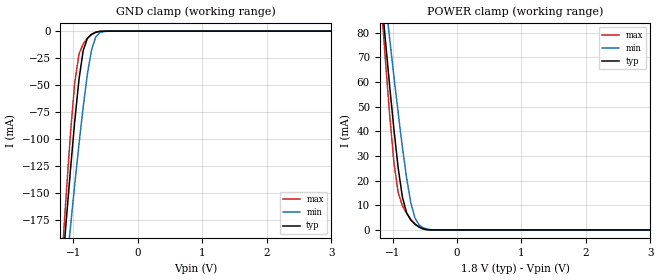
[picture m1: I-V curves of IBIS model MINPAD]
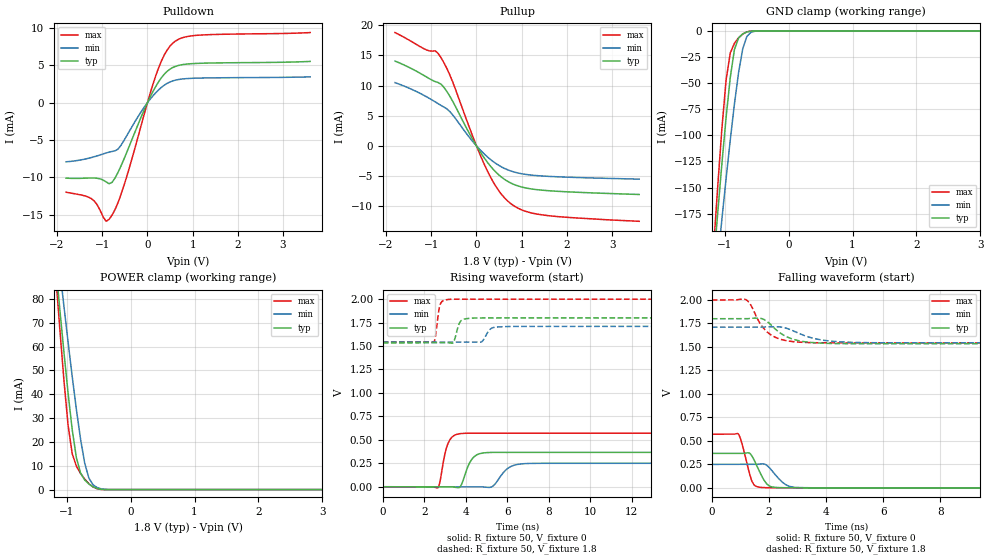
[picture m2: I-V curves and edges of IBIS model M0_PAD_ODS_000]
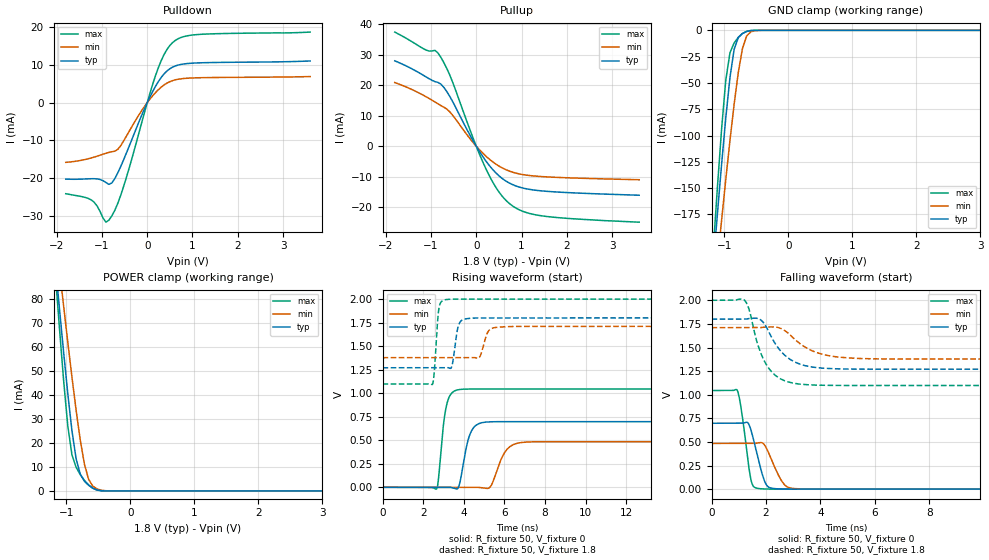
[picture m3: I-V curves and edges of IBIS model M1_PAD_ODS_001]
|   Microsemi Corporation
|   SmartFusion2 Automotive IBIS Model
[IBIS ver]   5.0
[File name]   as30208cc_18v_rev2p12.ibs
[File Rev]   2.12
[Date]   Wed Apr 02 2025
[Source] Simulated Models ONLY.
   All data is based on Spice simulation. All performed at Microsemi Corporation.
   Please refer to the Microsemi website for future updates at www.microsemi.com
[Notes]  Microsemi SmartFusion2 IBIS models for automotive operating conditions
   for DDRIO IO Banks IO Configurations ONLY. Models uses a software default
   fixed codes except for DDR3/SSTL15 which will always require calibrated
   codes.
   Automotive Temperature Grade 2 (t2) models cover a temperature range from
   -40C to 125C.
   Please refer to msio_auto_t2.ibs for MSIO IO Banks IO Configurations.
   Please refer to msiod_auto_t2.ibs for MSIOD IO Banks IO Configurations.
   The package parasitics of various package types are given.
   Uncomment the appropriate package or refer to the .pkg for specific
   per pin parasitic data.
   There are warnings related to non-monotonic and Increasing/Decreasing Current.
   They are expected on 20 Ohms and 30 Ohms I/O ODT models in DDR3/SSTL15.
[Disclaimer] This information is for board design considerations.
   Simulation based V/I curves contained in this model file are
   considered preliminary until verified against bench
   measurements. Maximum currents may vary from part to part but
   should not exceed maximum I/V curves provided in this model file.
[Copyright]  (c) 2015, Microsemi Corporation, All Rights Reserved.
| IBIS MODEL CHECKLIST
| Microsemi is dedicated to releasing quality IBIS models to customers.
| The following items have been
| verified for this IBIS model before release:
| 1)  Checked IBIS model by the golden parser ibischk5 [Complete]
| 2)  Ensured no errors reported by golden parser
|   for the IBIS model [Complete]
| 3)  Defined Vinl and Vinh for recievers [Complete]
| 4)  Defined Standard Load and Vmeas values for drivers [Complete]
| 5)  Defined overshoots for drivers and recievers [NA]
| 6)  Validated Ramp Values[Complete]
| 7)  Defined V-T Tables for all output drivers [Complete]
| 8)  Validated [Diff Pins] []
| 9)  Verified Package Parasitics [Complete]
| 10) Defined Standard Load Parameters and Specifications
|   for waveforms [Complete]
| 11) Defined and Validate Pin mappings [Complete]
| 12) Verified Ccomp Value []
| 13) Visually Inspected I-V Curves and V-T Tables  [Complete]
| 14) Presented Typ/Min/Max Values in the correct order for
|   all tables and parameters [Complete]
| 15) Simulated all output models with standard load and
|   switching through Vmeas [Complete]
| 16) Simulated all reciever models  [Complete]
| 17) Validated Models selectors. []
| 18) Visually inspected Spice and IBIS correlation for
|   a) Typical VT Curves [Complete]
|   b) Minimum VT Curves [Complete]
|   c) Maximum VT Curves [Complete]
| 19) Visually inspected Silicon and IBIS correlation
|   a) Typical IV Pull UP/ Pull Down Curves []
|   b) Minimum IV Pull UP/ Pull Down Curves []
|   c) Maximum IV Pull UP/ Pull Down Curves []
|   Component SmartFusion2
[Component]   SmartFusion2 W MRAM
[Manufacturer]   Avalanche Technology
[Package]
|  Design die-package: BGA
| variable   typ   min   max
R_pkg   0.72029   0.51528   1.0002
L_pkg   5.797e-9   4.155e-9   8.073e-9
C_pkg   1.116e-12   7.907e-13   1.753e-12
|Pin and Model info
[Pin]  signal_name  model_name   R_pin   L_pin   C_pin
L7   CS1#   MINPAD   0.4340		15.2000E-9		1.2600E-12
J8   CS2#   MINPAD   0.3800		13.5000E-9		1.0400E-12
K7   CLK1   MINPAD   0.4300		12.7000E-9		0.9790E-12
K6   CLK2   MINPAD   0.4480		14.6000E-9		1.1600E-12
M8   IO_0   MIOPAD   0.4010		12.4000E-9		1.2500E-12
M7   IO_1   MIOPAD   0.4050		14.2000E-9		1.1100E-12
L9   IO_2   MIOPAD   0.3780		11.8000E-9		1.2000E-12
M9   IO_3   MIOPAD   0.3700		11.8000E-9		1.2600E-12
M10   IO_4   MIOPAD   0.3710		11.1000E-9		1.1000E-12
N8   IO_5   MIOPAD   0.4050		13.8000E-9		1.1600E-12
N7   IO_6   MIOPAD   0.3830		15.2000E-9		1.0900E-12
N6   IO_7   MIOPAD   0.4480		16.4000E-9		1.0800E-12
J12   HTBSEL   MINPAD   0.1380		6.1700E-9		0.6060E-12
H12   HBP_2   MINPAD   0.1470		6.3900E-9		1.0000E-12
G11   HBP_1   MINPAD   0.1910		8.5000E-9		1.1500E-12
G10   HBP_0   MINPAD   0.2050		8.6800E-9		1.4200E-12
J9   RESET#   MINPAD   0.3410		14.1000E-9		1.6300E-12
J10   INT1#   MIOPAD   0.3080		12.5000E-9		1.2100E-12
K8   INT2#   MIOPAD   0.2120		10.3000E-9		0.8230E-12
M5   VSSIO   GND   NA   NA   NA
H6   VSSIO   GND   NA   NA   NA
L6   VSSIO   GND   NA   NA   NA
P8   VSSIO   GND   NA   NA   NA
H10   VSSIO   GND   NA   NA   NA
N10   VSSIO   GND   NA   NA   NA
P10   VSSIO   GND   NA   NA   NA
H11   VSSIO   GND   NA   NA   NA
N11   VSSIO   GND   NA   NA   NA
A1   VSS   GND   NA   NA   NA
B1   VSS   GND   NA   NA   NA
W1   VSS   GND   NA   NA   NA
Y1   VSS   GND   NA   NA   NA
A2   VSS   GND   NA   NA   NA
Y2   VSS   GND   NA   NA   NA
F3   VSS   GND   NA   NA   NA
G3   VSS   GND   NA   NA   NA
P3   VSS   GND   NA   NA   NA
R3   VSS   GND   NA   NA   NA
F4   VSS   GND   NA   NA   NA
H4   VSS   GND   NA   NA   NA
J4   VSS   GND   NA   NA   NA
L4   VSS   GND   NA   NA   NA
N4   VSS   GND   NA   NA   NA
R4   VSS   GND   NA   NA   NA
L5   VSS   GND   NA   NA   NA
N5   VSS   GND   NA   NA   NA
G6   VSS   GND   NA   NA   NA
P6   VSS   GND   NA   NA   NA
G8   VSS   GND   NA   NA   NA
H8   VSS   GND   NA   NA   NA
L10   VSS   GND   NA   NA   NA
L11   VSS   GND   NA   NA   NA
P11   VSS   GND   NA   NA   NA
F12   VSS   GND   NA   NA   NA
L12   VSS   GND   NA   NA   NA
N12   VSS   GND   NA   NA   NA
R12   VSS   GND   NA   NA   NA
F13   VSS   GND   NA   NA   NA
G13   VSS   GND   NA   NA   NA
P13   VSS   GND   NA   NA   NA
R13   VSS   GND   NA   NA   NA
A14   VSS   GND   NA   NA   NA
Y14   VSS   GND   NA   NA   NA
A15   VSS   GND   NA   NA   NA
B15   VSS   GND   NA   NA   NA
W15   VSS   GND   NA   NA   NA
Y15   VSS   GND   NA   NA   NA
G4   VCCIO   POWER   NA   NA   NA
P4   VCCIO   POWER   NA   NA   NA
G5   VCCIO   POWER   NA   NA   NA
J5   VCCIO   POWER   NA   NA   NA
P5   VCCIO   POWER   NA   NA   NA
M6   VCCIO   POWER   NA   NA   NA
H7   VCCIO   POWER   NA   NA   NA
H9   VCCIO   POWER   NA   NA   NA
N9   VCCIO   POWER   NA   NA   NA
J11   VCCIO   POWER   NA   NA   NA
M11   VCCIO   POWER   NA   NA   NA
G12   VCCIO   POWER   NA   NA   NA
P12   VCCIO   POWER   NA   NA   NA
K4   VCC   POWER   NA   NA   NA
M4   VCC   POWER   NA   NA   NA
K5   VCC   POWER   NA   NA   NA
G7   VCC   POWER   NA   NA   NA
P7   VCC   POWER   NA   NA   NA
G9   VCC   POWER   NA   NA   NA
K9   VCC   POWER   NA   NA   NA
P9   VCC   POWER   NA   NA   NA
K11   VCC   POWER   NA   NA   NA
K12   VCC   POWER   NA   NA   NA
M12   VCC   POWER   NA   NA   NA
| END PIN INFO
| IOPAD
[Model Selector] MIOPAD
| Model Description
M0_PAD_ODS_000   ODS_000
M1_PAD_ODS_001   ODS_001
M2_PAD_ODS_010   ODS_010
M3_PAD_ODS_011   ODS_011
M4_PAD_ODS_100   ODS_100
M5_PAD_ODS_101   ODS_101
M6_PAD_ODS_110   ODS_110
M7_PAD_ODS_111   ODS_111
| Models and submodels in the file (9): MINPAD (Input), M0_PAD_ODS_000 (I/O), M1_PAD_ODS_001 (I/O), M2_PAD_ODS_010 (I/O), M3_PAD_ODS_011 (I/O), M4_PAD_ODS_100 (I/O), M5_PAD_ODS_101 (I/O), M6_PAD_ODS_110 (I/O), M7_PAD_ODS_111 (I/O)
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[Model] MINPAD
Model_type Input
Enable   Active-High
Vinl  =  0.63
Vinh  =  1.17
| Capacitance  typ   min   max
C_comp   1.624351e-12   1.517192e-12   1.739751e-12
| Variables   typ   min   max
[GND Clamp Reference]   0   0   0
[POWER Clamp Reference]   1.8   1.71   2
[Pulldown Reference]   0   0   0
[Pullup Reference]   1.8   1.71   2
[Temperature Range]   25   125   -40
[Voltage Range]   1.8   1.71   2
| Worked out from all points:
|   GND clamp passes 1 mA (typ) near -0.64 V on its own axis
|   POWER clamp passes 1 mA (typ) near -0.57 V on its own axis
[GND Clamp]
| Voltage   I(typ)   I(min)   I(max)
-1.8V     -720.5mA   -670.5mA   -825.4mA
-1.173V   -222.3mA   -260.3mA   -207.7mA
-1.108V   -173.8mA   -219.8mA   -148.5mA
-1.043V   -127mA     -180.1mA   -93.29mA
-977.6mV  -83.06mA   -141.5mA   -47.18mA
-912.4mV  -44.72mA   -104.6mA   -21.22mA
-847.2mV  -17.98mA   -70.1mA    -11.91mA
-782.1mV  -6.764mA   -39.85mA   -6.651mA
-716.9mV  -2.937mA   -17.13mA   -3.044mA
-651.7mV  -1.118mA   -5.25mA    -949.8uA
-456.2mV  -3.975uA   -74.4uA    -419.6nA
3.6V      0A         0A         0A
[POWER Clamp]
| Voltage   I(typ)   I(min)   I(max)
-1.8V     287.1mA    268.3mA    329.6mA
-1.173V   94.89mA    108.5mA    91.02mA
-1.108V   76.1mA     92.66mA    67.97mA
-1.043V   57.9mA     77.16mA    46.14mA
-977.6mV  40.62mA    62.05mA    27.14mA
-912.4mV  25.13mA    47.46mA    15.06mA
-847.2mV  13.38mA    33.64mA    9.853mA
-716.9mV  4.014mA    11.09mA    4.394mA
-651.7mV  2.34mA     4.821mA    2.483mA
-586.6mV  1.18mA     2.003mA    1.113mA
-325.9mV  1.153uA    19.85uA    110.1nA
3.6V      0A         0A         0A
[Model] M0_PAD_ODS_000
Model_type I/O
Enable   Active-High
Vinl  =  0.63
Vinh  =  1.17
Vmeas =  0.9
Cref  =  30e-12
| Capacitance  typ   min   max
C_comp   1.627116e-12   1.521588e-12   1.744735e-12
| Variables   typ   min   max
[GND Clamp Reference]   0   0   0
[POWER Clamp Reference]   1.8   1.71   2
[Pulldown Reference]   0   0   0
[Pullup Reference]   1.8   1.71   2
[Temperature Range]   25   125   -40
[Voltage Range]   1.8   1.71   2
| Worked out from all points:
|   slope of the pulldown table from 0 to 0.27 V, typ, clamps not added: 89.8 ohm
|   slope of the pullup table from 0 to 0.27 V, typ, clamps not added: 90.4 ohm
|   GND clamp passes 1 mA (typ) near -0.64 V on its own axis
|   POWER clamp passes 1 mA (typ) near -0.57 V on its own axis
|   falling waveform, R_fixture 50, V_fixture 0: 20-80 % time 364ps typ, 459ps min, 289ps max; typ from 0.367 V to 0 V
|   falling waveform, R_fixture 50, V_fixture 1.8: 20-80 % time 770ps typ, 991ps min, 610ps max; typ from 1.8 V to 1.53 V
|   rising waveform, R_fixture 50, V_fixture 0: 20-80 % time 416ps typ, 570ps min, 332ps max; typ from 0 V to 0.367 V
|   rising waveform, R_fixture 50, V_fixture 1.8: 20-80 % time 213ps typ, 281ps min, 164ps max; typ from 1.53 V to 1.8 V
[GND Clamp]
| Voltage   I(typ)   I(min)   I(max)
-1.8V     -720.5mA   -670.5mA   -825.4mA
-1.173V   -222.3mA   -260.3mA   -207.7mA
-1.108V   -173.8mA   -219.8mA   -148.5mA
-1.043V   -127mA     -180.1mA   -93.3mA
-977.6mV  -83.06mA   -141.5mA   -47.19mA
-912.4mV  -44.72mA   -104.6mA   -21.23mA
-847.2mV  -17.99mA   -70.1mA    -11.92mA
-782.1mV  -6.766mA   -39.85mA   -6.657mA
-716.9mV  -2.938mA   -17.13mA   -3.048mA
-651.7mV  -1.119mA   -5.25mA    -952uA
-456.2mV  -3.98uA    -74.41uA   -422.2nA
3.6V      0A         0A         0A
[POWER Clamp]
| Voltage   I(typ)   I(min)   I(max)
-1.8V     287.1mA    268.3mA    329.6mA
-1.173V   94.89mA    108.5mA    91.02mA
-1.108V   76.1mA     92.66mA    67.97mA
-1.043V   57.9mA     77.16mA    46.14mA
-977.6mV  40.62mA    62.05mA    27.14mA
-912.4mV  25.13mA    47.46mA    15.06mA
-847.2mV  13.38mA    33.64mA    9.853mA
-716.9mV  4.014mA    11.09mA    4.394mA
-651.7mV  2.34mA     4.821mA    2.483mA
-586.6mV  1.18mA     2.003mA    1.113mA
-325.9mV  1.153uA    19.85uA    110.1nA
3.6V      0A         0A         0A
[Pulldown]
| Voltage   I(typ)   I(min)   I(max)
-1.8V     -10.09mA   -7.898mA   -11.97mA
-1.238V   -10.07mA   -7.328mA   -12.83mA
-912.4mV  -10.59mA   -6.717mA   -15.86mA
-847.2mV  -10.83mA   -6.605mA   -15.6mA
-716.9mV  -10.08mA   -6.431mA   -14.3mA
-521.4mV  -7.575mA   -5.077mA   -11.12mA
-65.17mV  -872uA     -545.4uA   -1.404mA
248.3mV   2.817mA    1.73mA     4.683mA
434.5mV   4.193mA    2.586mA    7.041mA
620.7mV   4.869mA    3.026mA    8.258mA
1.179V    5.284mA    3.307mA    9.058mA
3.6V      5.531mA    3.462mA    9.391mA
[Pullup]
| Voltage   I(typ)   I(min)   I(max)
-1.8V     14.07mA    10.49mA    18.8mA
-1.108V   11.45mA    8.161mA    15.93mA
-912.4mV  10.66mA    7.301mA    15.78mA
-782.1mV  10.22mA    6.706mA    14.62mA
-586.6mV  8.214mA    5.673mA    11.74mA
-65.17mV  835.7uA    571.5uA    1.251mA
248.3mV   -2.782mA   -1.866mA   -4.251mA
496.6mV   -4.831mA   -3.242mA   -7.473mA
744.8mV   -6.111mA   -4.126mA   -9.499mA
1.055V    -6.927mA   -4.698mA   -10.78mA
1.428V    -7.337mA   -4.986mA   -11.42mA
3.6V      -8.069mA   -5.52mA    -12.52mA
[Ramp]
dV/dt_r   0.220223/0.415702n  0.150081/0.569672n  0.34276/0.331988n
dV/dt_f   0.159898/0.770039n  0.100158/0.991323n  0.274318/0.609698n
R_load = 50
[Falling Waveform]
R_fixture = 50
V_fixture = 0
V_fixture_min = 0
V_fixture_max = 0
| Time   V(typ)   V(min)   V(max)
0s        367mV      250.1mV    571.3mV
923.8ps   367.3mV    250.7mV    573.7mV
1.037ns   367.3mV    250.7mV    489.3mV
1.291ns   372.9mV    250.9mV    184mV
1.42ns    330.5mV    250.9mV    60.14mV
1.744ns   128.3mV    254.8mV    4.316mV
2.055ns   13.67mV    200.4mV    1.169mV
2.601ns   1.34mV     30.95mV    220.5uV
2.98ns    480.5uV    4.171mV    216.1uV
21.88ns   3.869uV    78.26nV    -3.43uV
[Falling Waveform]
R_fixture = 50
V_fixture = 1.8
V_fixture_min = 1.71
V_fixture_max = 2
| Time   V(typ)   V(min)   V(max)
0s        1.8V       1.71V      2V
1.194ns   1.801V     1.71V      2.003V
1.367ns   1.805V     1.71V      1.943V
1.68ns    1.806V     1.711V     1.755V
1.949ns   1.766V     1.714V     1.656V
2.444ns   1.638V     1.711V     1.578V
2.887ns   1.578V     1.666V     1.554V
3.81ns    1.541V     1.576V     1.544V
5.079ns   1.534V     1.547V     1.543V
21.88ns   1.534V     1.543V     1.543V
[Rising Waveform]
R_fixture = 50
V_fixture = 0
V_fixture_min = 0
V_fixture_max = 0
| Time   V(typ)   V(min)   V(max)
0s        3.036nV    85.33nV    -62.8nV
2.644ns   -691.4uV   -545.1uV   -11.75mV
3.145ns   -822.4uV   -648.4uV   462.5mV
3.72ns    -1.25mV    -766.9uV   565.8mV
4.314ns   300mV      -889.5uV   570.7mV
5.019ns   364.1mV    -5.657mV   570.7mV
5.313ns   366.1mV    6.668mV    570.7mV
6.157ns   366.1mV    214mV      570.8mV
6.888ns   366.1mV    247mV      570.8mV
21.88ns   367mV      250.1mV    571.3mV
[Rising Waveform]
R_fixture = 50
V_fixture = 1.8
V_fixture_min = 1.71
V_fixture_max = 2
| Time   V(typ)   V(min)   V(max)
0s        1.534V     1.543V     1.543V
2.445ns   1.534V     1.543V     1.54V
2.53ns    1.534V     1.543V     1.594V
2.745ns   1.534V     1.543V     1.929V
3.139ns   1.534V     1.543V     1.996V
3.396ns   1.538V     1.543V     1.999V
3.757ns   1.766V     1.543V     1.999V
4.265ns   1.797V     1.543V     1.999V
5.688ns   1.8V       1.705V     1.999V
21.88ns   1.8V       1.71V      2V
[Model] M1_PAD_ODS_001
Model_type I/O
Enable   Active-High
Vinl  =  0.63
Vinh  =  1.17
Vmeas =  0.9
Cref  =  30e-12
| Capacitance  typ   min   max
C_comp   1.627116e-12   1.521588e-12   1.744735e-12
| Variables   typ   min   max
[GND Clamp Reference]   0   0   0
[POWER Clamp Reference]   1.8   1.71   2
[Pulldown Reference]   0   0   0
[Pullup Reference]   1.8   1.71   2
[Temperature Range]   25   125   -40
[Voltage Range]   1.8   1.71   2
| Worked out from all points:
|   slope of the pulldown table from 0 to 0.27 V, typ, clamps not added: 44.9 ohm
|   slope of the pullup table from 0 to 0.27 V, typ, clamps not added: 45.3 ohm
|   GND clamp passes 1 mA (typ) near -0.64 V on its own axis
|   POWER clamp passes 1 mA (typ) near -0.57 V on its own axis
|   falling waveform, R_fixture 50, V_fixture 0: 20-80 % time 370ps typ, 463ps min, 286ps max; typ from 0.698 V to 0 V
|   falling waveform, R_fixture 50, V_fixture 1.8: 20-80 % time 821ps typ, 1.04ns min, 652ps max; typ from 1.8 V to 1.27 V
|   rising waveform, R_fixture 50, V_fixture 0: 20-80 % time 411ps typ, 571ps min, 311ps max; typ from 0 V to 0.698 V
|   rising waveform, R_fixture 50, V_fixture 1.8: 20-80 % time 216ps typ, 282ps min, 166ps max; typ from 1.27 V to 1.8 V
[GND Clamp]
| Voltage   I(typ)   I(min)   I(max)
-1.8V     -720.5mA   -670.5mA   -825.4mA
-1.173V   -222.3mA   -260.3mA   -207.7mA
-1.108V   -173.8mA   -219.8mA   -148.5mA
-1.043V   -127mA     -180.1mA   -93.3mA
-977.6mV  -83.06mA   -141.5mA   -47.19mA
-912.4mV  -44.72mA   -104.6mA   -21.23mA
-847.2mV  -17.99mA   -70.1mA    -11.92mA
-782.1mV  -6.766mA   -39.85mA   -6.657mA
-716.9mV  -2.938mA   -17.13mA   -3.048mA
-651.7mV  -1.119mA   -5.25mA    -952uA
-456.2mV  -3.98uA    -74.41uA   -422.2nA
3.6V      0A         0A         0A
[POWER Clamp]
| Voltage   I(typ)   I(min)   I(max)
-1.8V     287.1mA    268.3mA    329.6mA
-1.173V   94.89mA    108.5mA    91.02mA
-1.108V   76.1mA     92.66mA    67.97mA
-1.043V   57.9mA     77.16mA    46.14mA
-977.6mV  40.62mA    62.05mA    27.14mA
-912.4mV  25.13mA    47.46mA    15.06mA
-847.2mV  13.38mA    33.64mA    9.853mA
-716.9mV  4.014mA    11.09mA    4.394mA
-651.7mV  2.34mA     4.821mA    2.483mA
-586.6mV  1.18mA     2.003mA    1.113mA
-325.9mV  1.153uA    19.85uA    110.1nA
3.6V      0A         0A         0A
[Pulldown]
| Voltage   I(typ)   I(min)   I(max)
-1.8V     -20.26mA   -15.83mA   -24.15mA
-1.238V   -20.17mA   -14.67mA   -25.78mA
-912.4mV  -21.17mA   -13.42mA   -31.69mA
-847.2mV  -21.66mA   -13.2mA    -31.16mA
-716.9mV  -20.14mA   -12.86mA   -28.56mA
-521.4mV  -15.14mA   -10.15mA   -22.2mA
-65.17mV  -1.742mA   -1.091mA   -2.802mA
248.3mV   5.63mA     3.46mA     9.353mA
434.5mV   8.383mA    5.171mA    14.07mA
620.7mV   9.735mA    6.051mA    16.51mA
1.179V    10.57mA    6.614mA    18.12mA
3.6V      11.06mA    6.923mA    18.71mA
[Pullup]
| Voltage   I(typ)   I(min)   I(max)
-1.8V     28.03mA    20.89mA    37.45mA
-1.108V   22.74mA    16.24mA    31.55mA
-912.4mV  21.2mA     14.52mA    31.47mA
-782.1mV  20.39mA    13.35mA    29.17mA
-521.4mV  14.66mA    10.17mA    21.02mA
-130.3mV  3.403mA    2.332mA    5.058mA
186.2mV   -4.285mA   -2.877mA   -6.521mA
496.6mV   -9.629mA   -6.461mA   -14.9mA
744.8mV   -12.18mA   -8.22mA    -18.94mA
1.055V    -13.81mA   -9.36mA    -21.49mA
1.49V     -14.71mA   -9.993mA   -22.92mA
3.6V      -16.07mA   -10.99mA   -24.92mA
[Ramp]
dV/dt_r   0.418626/0.410816n  0.290552/0.571412n  0.626829/0.311374n
dV/dt_f   0.317973/0.820722n  0.199636/1.04338n  0.541445/0.651669n
R_load = 50
[Falling Waveform]
R_fixture = 50
V_fixture = 0
V_fixture_min = 0
V_fixture_max = 0
| Time   V(typ)   V(min)   V(max)
0s        697.7mV    484.3mV    1.045V
951.4ps   698.1mV    484.5mV    1.042V
1.108ns   698.1mV    484.5mV    814.4mV
1.331ns   703.6mV    484.6mV    322mV
1.452ns   622mV      484.6mV    93.29mV
1.73ns    303.2mV    490.6mV    6.618mV
2.068ns   27.7mV     403mV      1.399mV
2.572ns   2.158mV    87.65mV    450.6uV
3.037ns   658.8uV    6.568mV    439.8uV
21.88ns   1.498nV    129.2nV    255.6nV
[Falling Waveform]
R_fixture = 50
V_fixture = 1.8
V_fixture_min = 1.71
V_fixture_max = 2
| Time   V(typ)   V(min)   V(max)
0s        1.8V       1.71V      2V
1.215ns   1.801V     1.71V      2V
1.378ns   1.807V     1.71V      1.904V
1.7ns     1.808V     1.71V      1.529V
1.992ns   1.728V     1.717V     1.329V
2.553ns   1.458V     1.701V     1.165V
3.071ns   1.345V     1.583V     1.119V
4.039ns   1.282V     1.431V     1.1V
5.423ns   1.271V     1.384V     1.098V
21.88ns   1.27V      1.377V     1.098V
[Rising Waveform]
R_fixture = 50
V_fixture = 0
V_fixture_min = 0
V_fixture_max = 0
| Time   V(typ)   V(min)   V(max)
0s        2.474nV    66.45nV    166.5nV
2.668ns   -425.3uV   -220uV     -14.74mV
3.141ns   -500.7uV   -259uV     861mV
3.645ns   -17.16mV   -300.5uV   1.033V
4.267ns   540.5mV    -351.8uV   1.044V
4.874ns   685.9mV    -4.978mV   1.044V
5.31ns    695.8mV    6.141mV    1.044V
6.12ns    697mV      401.5mV    1.044V
6.901ns   697.1mV    477.2mV    1.044V
21.88ns   697.7mV    484.3mV    1.045V
[Rising Waveform]
R_fixture = 50
V_fixture = 1.8
V_fixture_min = 1.71
V_fixture_max = 2
| Time   V(typ)   V(min)   V(max)
0s        1.27V      1.377V     1.098V
2.449ns   1.271V     1.378V     1.092V
2.769ns   1.271V     1.378V     1.892V
3.098ns   1.271V     1.378V     1.993V
3.393ns   1.274V     1.378V     1.999V
3.717ns   1.703V     1.378V     2V
4.17ns    1.792V     1.378V     2V
4.743ns   1.799V     1.375V     2V
5.693ns   1.799V     1.701V     2V
21.88ns   1.8V       1.71V      2V
